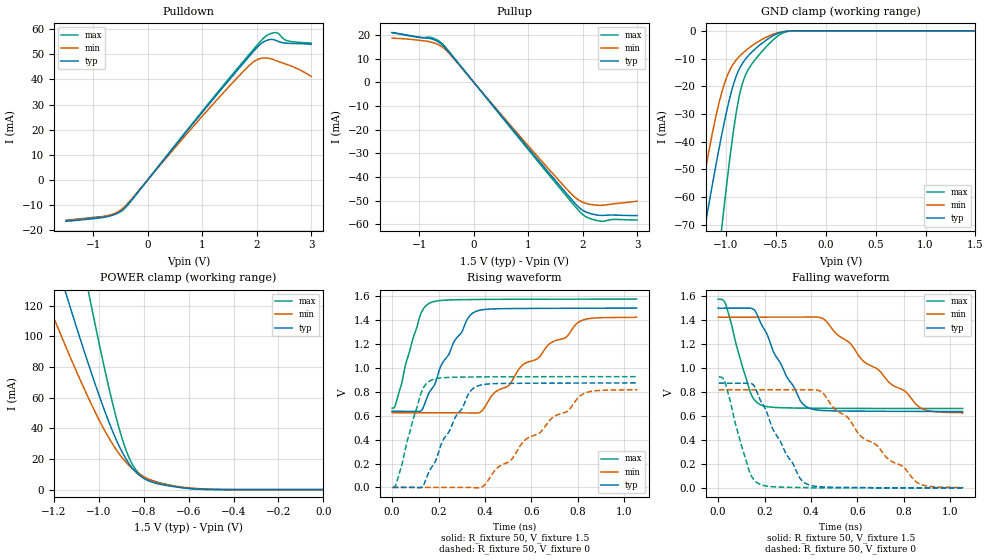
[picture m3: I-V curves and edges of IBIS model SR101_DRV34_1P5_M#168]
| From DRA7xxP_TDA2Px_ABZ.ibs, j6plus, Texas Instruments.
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| Model based on original model for DDR_DIFFIOPB_H
|   Sub model SR101_DRV34_1P5
[model]   SR101_DRV34_1P5_M#168
|[Description]  [1.5V-I/O-X-X]
|   , ,
|[Input Load]
|[Output Drive]
|Voltage   1.5V
|Mode   I/O
Model_type   I/O
Polarity   Non-Inverting
Enable   Active-Low
Vinl =  0.65
Vinh =  0.85
Cref =  15.0000pF
Rref =  100.0000M
Vref =  0V
Vmeas =  0.75
C_comp   2p   2p   2p
[Model Spec]
Vinl   0.65   0.6125   0.6875
Vinh   0.85   0.8125   0.8875
[Receiver Thresholds]
Tslew_ac = 0.5n
Vth = 0.75
Vth_max = 0.7875
Vth_min = 0.675
Vinh_ac = 0.175
Vinh_dc = 0.1
Vinl_ac = -0.175
Vinl_dc = -0.1
[Temperature Range]   25   125   -40
[Voltage Range]   1.5   1.425   1.575
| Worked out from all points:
|   slope of the pulldown table from 0 to 0.225 V, typ, clamps not added: 36.8 ohm
|   slope of the pullup table from 0 to 0.225 V, typ, clamps not added: 35.8 ohm
|   GND clamp passes 1 mA (typ) near -0.48 V on its own axis
|   POWER clamp passes 1 mA (typ) near -0.62 V on its own axis
|   rising waveform, R_fixture 50, V_fixture 1.5: 20-80 % time 141ps typ, 317ps min, 75.9ps max; typ from 0.637 V to 1.5 V
|   rising waveform, R_fixture 50, V_fixture 0: 20-80 % time 139ps typ, 311ps min, 75.5ps max; typ from 0 V to 0.874 V
|   falling waveform, R_fixture 50, V_fixture 1.5: 20-80 % time 137ps typ, 294ps min, 76.5ps max; typ from 1.5 V to 0.637 V
|   falling waveform, R_fixture 50, V_fixture 0: 20-80 % time 138ps typ, 300ps min, 76.4ps max; typ from 0.874 V to 0 V
[POWER_clamp]
-1.5V     302.8mA    223.9mA    484.4mA
-1.242V   174.3mA    127.3mA    279.1mA
-1.136V   123.3mA    89.68mA    196.8mA
-1.045V   81.65mA    59.62mA    128.8mA
-1.03V    75mA       54.92mA    117.8mA
-939.4mV  38.44mA    29.91mA    56.84mA
-893.9mV  23.93mA    20.41mA    32.31mA
-848.5mV  13.61mA    13.43mA    15.91mA
-803mV    7.623mA    8.663mA    8.564mA
-712.1mV  3.022mA    3.561mA    3.877mA
-575.8mV  470.5uA    872uA      449uA
0V        112.6nA    435.6nA    613.8nA
[Pulldown]
-1.5V     -16.54mA   -16.32mA   -16.11mA
-727.3mV  -14.62mA   -14.26mA   -14.29mA
-545.5mV  -13.24mA   -12.72mA   -13.05mA
-409.1mV  -10.94mA   -10.36mA   -11.07mA
1.227V    32.84mA    30.87mA    33.41mA
1.818V    48.09mA    44.61mA    48.84mA
2V        52.62mA    47.82mA    53.46mA
2.182V    55.55mA    48.58mA    57.5mA
2.273V    55.99mA    48.2mA     58.42mA
2.364V    55.5mA     47.46mA    58.71mA
2.545V    54.48mA    46.06mA    55.55mA
3V        54mA       41.23mA    54.49mA
[Pullup]
-1.5V     20.96mA    18.6mA     20.95mA
-1V       19mA       17.69mA    18.93mA
-772.7mV  18.26mA    16.89mA    18.84mA
-590.9mV  16.04mA    15.07mA    16.54mA
-409.1mV  11.43mA    11.07mA    11.7mA
1.409V    -38.97mA   -37.46mA   -39.88mA
1.773V    -48.83mA   -46.66mA   -49.96mA
1.909V    -52.33mA   -49.44mA   -53.68mA
2.045V    -54.57mA   -50.97mA   -56.55mA
2.273V    -56.03mA   -51.89mA   -58.38mA
2.591V    -56.03mA   -51.23mA   -57.86mA
3V        -56.26mA   -50.14mA   -58.12mA
[GND_clamp]
-1.5V     -133.6mA   -115.7mA   -234.3mA
-1.288V   -87.29mA   -67.59mA   -156.8mA
-1.197V   -68.11mA   -48.64mA   -124.4mA
-1.045V   -38.25mA   -22.77mA   -72.51mA
-1.015V   -32.88mA   -19.1mA    -62.74mA
-954.5mV  -23.3mA    -13.72mA   -44.4mA
-863.6mV  -13.6mA    -9.192mA   -23.11mA
-803mV    -10.18mA   -7.193mA   -15.89mA
-681.8mV  -5.771mA   -4.027mA   -9.287mA
-500mV    -1.264mA   -914.7uA   -2.429mA
-348.5mV  -52.39uA   -75.11uA   -85.87uA
1.5V      112.6nA    528.1nA    514.5nA
[Ramp]
dV/dt_f 0.51826109/0.13691342n  0.4815074/0.29468571n 0.54809736/76.538797p
dV/dt_r 0.52631337/0.13946652n 0.49366604/0.31266692n  0.5577905/75.738849p
R_load = 50
[Rising Waveform]
R_fixture = 50
V_fixture = 1.5
V_fixture_min = 1.425
V_fixture_max = 1.575
0s        637.3mV    624.3mV    663.1mV
16.01ps   637.2mV    624.2mV    699.7mV
121.4ps   637.6mV    624.2mV    1.441V
164.8ps   808.6mV    624.2mV    1.545V
268.6ps   1.225V     624mV      1.569V
361ps     1.472V     621.8mV    1.572V
503.6ps   1.496V     855.4mV    1.574V
559.9ps   1.497V     1.02V      1.574V
805.9ps   1.499V     1.386V     1.575V
1.053ns   1.5V       1.425V     1.575V
[Rising Waveform]
R_fixture = 50
V_fixture = 0
V_fixture_min = 0
V_fixture_max = 0
2.65ps    0V         0V         0V
39.75ps   0V         0V         172.5mV
124.8ps   0V         0V         790.2mV
169ps     166.2mV    0V         897.4mV
273.3ps   590.9mV    0V         921.8mV
367.2ps   847.2mV    -3.707mV   924.3mV
511.4ps   870.5mV    227.3mV    925.8mV
571.4ps   871.4mV    394.5mV    926.1mV
818.9ps   873.2mV    777.5mV    926.6mV
1.055ns   874.1mV    819mV      926.7mV
[Falling Waveform]
R_fixture = 50
V_fixture = 1.5
V_fixture_min = 1.425
V_fixture_max = 1.575
0s        1.5V       1.425V     1.575V
31.67ps   1.5V       1.425V     1.537V
136.6ps   1.501V     1.425V     808.1mV
182.7ps   1.379V     1.425V     693.8mV
295.5ps   927.5mV    1.425V     667.8mV
388.5ps   668.5mV    1.426V     665.2mV
458.6ps   644.9mV    1.404V     664.1mV
623.3ps   640.2mV    1.062V     662.9mV
869.3ps   638.3mV    671mV      662.4mV
1.053ns   637.3mV    624.3mV    662.3mV
[Falling Waveform]
R_fixture = 50
V_fixture = 0
V_fixture_min = 0
V_fixture_max = 0
2.65ps    874.1mV    819mV      926.7mV
31.14ps   874.3mV    819.1mV    872.2mV
135.7ps   873.7mV    819.1mV    130.9mV
179ps     743.5mV    819mV      30.92mV
292.1ps   284.9mV    819mV      5.03mV
383.6ps   30.54mV    819.4mV    2.281mV
447.8ps   8.006mV    797.7mV    0V
614.6ps   2.564mV    430.3mV    0V
858.6ps   0V         42.93mV    0V
1.055ns   0V         0V         0V
